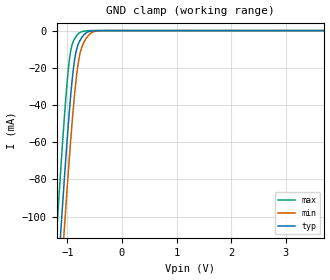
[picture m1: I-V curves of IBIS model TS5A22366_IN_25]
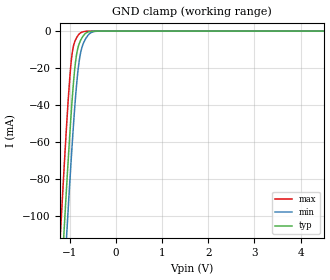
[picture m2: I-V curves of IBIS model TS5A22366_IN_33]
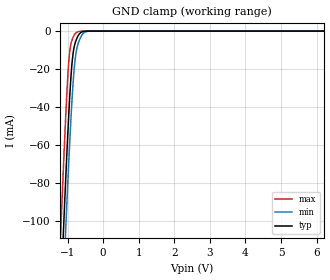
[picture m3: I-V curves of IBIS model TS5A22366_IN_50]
| TEXAS INSTRUMENTS INCORPORATED
| Standard Linear and Logic Group
| IBIS Model of TS5A22366
| 0.7-OHM DUAL SPDT ANALOG SWITCH WITH NEGATIVE RAIL CAPABILITY AND
| 1.8-V COMPATIBLE INPUT LOGIC
| This file contains package information for the following:
|  VSSOP 10-pin (RSE) package as [Component] TS5A22366_RSE
| This device can be powered at the following Vccs:
|  2.5 volt Vcc
|  3.3 volt Vcc
|  5 volt Vcc
| This file provides unique models under the [Model Selector] for each Vcc.
| For operation at a specific Vcc, select the appropriate model after each
| [Model Selector] keyword.
[IBIS Ver]   3.2
[Comment char]  |_char
[File Name]   ts5a22366.ibs
[File Rev]   1.0 | x_die
[Date]   March 22, 2009
[Source]   Data created from TI-SPICE simulations at TI-SLL.
[Notes]   The following is an IBIS list for the TS5A22366.
   Please contact sllibis@ti.com with questions and
   comments concerning SLL IBIS models.
   NOTE: No GND Clamp for switch, so that it can pass negative
   voltages.
   - FILE REV HISTORY
   - 1.0 Release IBIS file on 4/7/09.
   - Power clamp data deleted was deleted as there is no
   power-clamp diode.
   - Non-monotonic data due to FET characteristics.
[Disclaimer] Property of Texas Instruments Incorporated.  Unauthorized
   reproduction and/or distribution is strictly prohibited.
   This product is protected under copyright law.
   Created  2009, (C) Copyright  2009, Texas Instruments
   Incorporated, All Rights Reserved
   UNLESS THERE IS A SIGNED, WRITTEN AGREEMENT TO THE
   CONTRARY, TEXAS INSTRUMENTS (TI) IS PROVIDING THE IBIS
   MODELS  AND WITHOUT ANY WARRANTY, EXPRESSED OR
   IMPLIED.  TI assumes no liability for:
   1) the accuracy of the IBIS models provided to your
   company;
   2) the proper functioning of these IBIS Models in your
   design or for any resulting applications; or
   3) infringement of patents, copyrights or intellectual
   property rights resulting from your use of these IBIS
   models.
   TI provides IBIS Models as a service to our customers.
   You and your company shall not distribute, sell or give
   these models to anyone else without prior written
   permission from TI.
   TI reserves the right to make changes to our products or
   to discontinue any semiconductor product or service
   without notice, and advises our customers to obtain the
   latest version of relevant information to verify, before
   placing orders, that the information being relied on is
   current.
   Please be aware that your receipt and use of the IBIS
   information provided shall serve as acceptance of these
   terms and conditions.  If you do not accept these terms,
   you should return or destroy the IBIS models and any
   other accompanying information immediately.
| Component TS5A22366_RSE 10-PIN VSSOP
[Component]   TS5A22366_RSE
[Manufacturer]   Texas Instruments, Inc.
[Package]
|   typ   min   max
R_pkg   4.300e-02   4.100e-02   4.700e-02
L_pkg   2.235e-09   2.157e-09   2.339e-09
C_pkg   3.350e-13   3.080e-13   3.550e-13
[Pin]   signal_name   model_name   R_pin   L_pin   C_pin
1   IN1   TS5A22366_IN   4.700e-02   2.339e-09   3.100e-13
2   NO1   TS5A22366_N   4.300e-02   2.213e-09   3.550e-13
3   COM1   TS5A22366_COM   4.100e-02   2.157e-09   3.540e-13
4   NC1   TS5A22366_N   4.300e-02   2.213e-09   3.550e-13
5   VP   POWER   4.700e-02   2.339e-09   3.100e-13
6   NC2   TS5A22366_N   4.500e-02   2.284e-09   3.080e-13
7   COM2   TS5A22366_COM   4.100e-02   2.176e-09   3.500e-13
8   NO2   TS5A22366_N   4.100e-02   2.172e-09   3.500e-13
9   IN2   TS5A22366_IN   4.100e-02   2.176e-09   3.510e-13
10   GND   GND   4.500e-02   2.284e-09   3.080e-13
[Series Switch Groups]
| Function Group States
On  1 /   | NC1-NC2->COM1-COM2 IN1-IN2, LOW
   | COM1-COM2->NC1-NC2 IN1-IN2, LOW
On  2 /   | NO1-NO2->COM1-COM2 IN1-IN2, HIGH
   | COM1-COM2->NO1-NO2 IN1-IN2, HIGH
On  1 /   | IN1-IN2, LOW
Off 2 /   | IN1-IN2, HIGH
[Series Pin Mapping]   pin_2   model_name   function_table_group
4   3   TS5A22366_N_25_S   1
| 4   3   TS5A22366_N_33_S   1
| 4   3   TS5A22366_N_50_S   1
6   7   TS5A22366_N_25_S   1
| 6   7   TS5A22366_N_33_S   1
| 6   7   TS5A22366_N_50_S   1
3   4   TS5A22366_COM_25_S   1
| 3   4   TS5A22366_COM_33_S   1
| 3   4   TS5A22366_COM_50_S   1
7   6   TS5A22366_COM_25_S   1
| 7   6   TS5A22366_COM_33_S   1
| 7   6   TS5A22366_COM_50_S   1
2   3   TS5A22366_N_25_S   2
| 2   3   TS5A22366_N_33_S   2
| 2   3   TS5A22366_N_50_S   2
8   7   TS5A22366_N_25_S   2
| 8   7   TS5A22366_N_33_S   2
| 8   7   TS5A22366_N_50_S   2
3   2   TS5A22366_COM_25_S   2
| 3   2   TS5A22366_COM_33_S   2
| 3   2   TS5A22366_COM_50_S   2
7   8   TS5A22366_COM_25_S   2
| 7   8   TS5A22366_COM_33_S   2
| 7   8   TS5A22366_COM_50_S   2
| Model TS5A22366_IN
[Model Selector]   TS5A22366_IN
TS5A22366_IN_25   2.5 volt Vcc
TS5A22366_IN_33   3.3 volt Vcc
TS5A22366_IN_50   5 volt Vcc
| Model TS5A22366_COM
[Model Selector]   TS5A22366_COM
TS5A22366_COM_25   2.5 volt Vcc
TS5A22366_COM_33   3.3 volt Vcc
TS5A22366_COM_50   5 volt Vcc
| Model TS5A22366_COM_S
[Model Selector]   TS5A22366_COM_S
TS5A22366_COM_25_S   2.5 volt Vcc
TS5A22366_COM_33_S   3.3 volt Vcc
TS5A22366_COM_50_S   5 volt Vcc
| Model TS5A22366_N
[Model Selector]   TS5A22366_N
TS5A22366_N_25   2.5 volt Vcc
TS5A22366_N_33   3.3 volt Vcc
TS5A22366_N_50   5 volt Vcc
| Model TS5A22366_N_S
[Model Selector]   TS5A22366_N_S
TS5A22366_N_25_S   2.5 volt Vcc
TS5A22366_N_33_S   3.3 volt Vcc
TS5A22366_N_50_S   5 volt Vcc
[Model]   TS5A22366_COM_25_S
Model_type  Series_switch
| variable   typ   min   max
C_comp   0   0   0
[Temperature Range]   40   100   -40
| Ambient temperature   25   85   -40
[Voltage range]   2.5   2.3   2.7
[On]
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[Off]
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[Model]   TS5A22366_COM_33_S
Model_type  Series_switch
| variable   typ   min   max
C_comp   0   0   0
[Temperature Range]   40   100   -40
| Ambient temperature   25   85   -40
[Voltage range]   3.3   3   3.6
[On]
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[Off]
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[Model]   TS5A22366_COM_50_S
Model_type  Series_switch
| variable   typ   min   max
C_comp   0   0   0
[Temperature Range]   40   100   -40
| Ambient temperature   25   85   -40
[Voltage range]   5   4.5   5.5
[On]
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[Off]
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[Model]   TS5A22366_N_25_S
Model_type  Series_switch
| variable   typ   min   max
C_comp   0   0   0
[Temperature Range]   40   100   -40
| Ambient temperature   25   85   -40
[Voltage range]   2.5   2.3   2.7
[On]
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[Off]
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[Model]   TS5A22366_N_33_S
Model_type  Series_switch
| variable   typ   min   max
C_comp   0   0   0
[Temperature Range]   40   100   -40
| Ambient temperature   25   85   -40
[Voltage range]   3.3   3   3.6
[On]
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[Off]
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[Model]   TS5A22366_N_50_S
Model_type  Series_switch
| variable   typ   min   max
C_comp   0   0   0
[Temperature Range]   40   100   -40
| Ambient temperature   25   85   -40
[Voltage range]   5   4.5   5.5
[On]
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[Off]
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| Models and submodels in the file (15): TS5A22366_IN_25 (Input), TS5A22366_IN_33 (Input), TS5A22366_IN_50 (Input), TS5A22366_COM_25_S (Series_switch), TS5A22366_COM_25 (Terminator), TS5A22366_COM_33_S (Series_switch), TS5A22366_COM_33 (Terminator), TS5A22366_COM_50_S (Series_switch), TS5A22366_COM_50 (Terminator), TS5A22366_N_25_S (Series_switch), TS5A22366_N_25 (Terminator), TS5A22366_N_33_S (Series_switch), TS5A22366_N_33 (Terminator), TS5A22366_N_50_S (Series_switch), TS5A22366_N_50 (Terminator)
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[Model]   TS5A22366_IN_25
Model_type  Input
Vinl=0.65
Vinh=1.05
| variable   typ   min   max
C_comp   2.29pF   1.88pF   2.79pF
[Temperature Range]   40   100   -40
| Ambient temperature   25   85   -40
[Voltage range]   2.5   2.3   2.7
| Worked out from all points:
|   GND clamp passes 1 mA (typ) near -0.64 V on its own axis
[GND Clamp]
| TS5A22366_IN_25
|   Voltage   I(typ)   I(min)   I(max)
-2.5V     -779mA     -802.6mA   -750.6mA
-1.21V    -147.9mA   -175mA     -114.1mA
-1.185V   -136.5mA   -163.6mA   -102.6mA
-1.125V   -109.5mA   -136.5mA   -75.72mA
-1.055V   -79.15mA   -105.8mA   -46.21mA
-1V       -56.72mA   -82.65mA   -25.99mA
-955mV    -39.95mA   -64.64mA   -13.73mA
-865mV    -15.04mA   -33.13mA   -4.26mA
-765mV    -5.08mA    -11.91mA   -969.3uA
-625mV    -721.5uA   -2.983mA   -61.93uA
-440mV    -14.35uA   -139uA     -188.5nA
5V        502.2nA    605.2nA    422.7nA
[Model]   TS5A22366_IN_33
Model_type  Input
Vinl=0.65
Vinh=1.05
| variable   typ   min   max
C_comp   2.23pF   1.79pF   2.82pF
[Temperature Range]   40   100   -40
| Ambient temperature   25   85   -40
[Voltage range]   3.3   3   3.6
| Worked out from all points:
|   GND clamp passes 1 mA (typ) near -0.64 V on its own axis
[GND Clamp]
| TS5A22366_IN_33
|   Voltage   I(typ)   I(min)   I(max)
-3.3V     -1.181A    -1.203A    -1.155A
-1.21V    -147.9mA   -175mA     -114.1mA
-1.19V    -138.8mA   -165.9mA   -104.9mA
-1.12V    -107.3mA   -134.3mA   -73.53mA
-1.06V    -81.27mA   -108mA     -48.21mA
-950mV    -38.22mA   -62.71mA   -12.73mA
-855mV    -13.32mA   -30.21mA   -3.774mA
-800mV    -7.229mA   -17.21mA   -1.716mA
-740mV    -3.89mA    -9.301mA   -651.5uA
-595mV    -429.3uA   -2.027mA   -26.81uA
-405mV    -5.679uA   -67.72uA   -95.74nA
6.6V      662.9nA    799.1nA    558nA
[Model]   TS5A22366_IN_50
Model_type  Input
Vinl=0.65
Vinh=1.05
| variable   typ   min   max
C_comp   2.15pF   1.70pF   2.90pF
[Temperature Range]   40   100   -40
| Ambient temperature   25   85   -40
[Voltage range]   5   4.5   5.5
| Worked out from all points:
|   GND clamp passes 1 mA (typ) near -0.64 V on its own axis
[GND Clamp]
| TS5A22366_IN_50
|   Voltage   I(typ)   I(min)   I(max)
-5V       -2.042A    -2.059A    -2.021A
-1.19V    -138.8mA   -165.9mA   -104.9mA
-1.11V    -102.9mA   -129.9mA   -69.18mA
-1.06V    -81.27mA   -108mA     -48.21mA
-960mV    -41.72mA   -66.59mA   -14.82mA
-895mV    -21.59mA   -42.73mA   -6.039mA
-830mV    -9.948mA   -23.61mA   -2.712mA
-780mV    -5.912mA   -13.91mA   -1.237mA
-710mV    -2.707mA   -7.034mA   -396.9uA
-560mV    -224.9uA   -1.201mA   -9.216uA
-375mV    -2.486uA   -35.45uA   -71.12nA
10V       1.005uA    1.213uA    845.4nA
